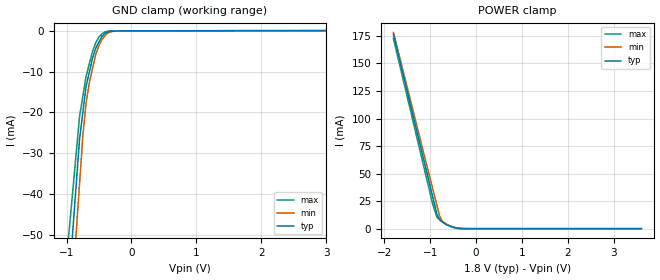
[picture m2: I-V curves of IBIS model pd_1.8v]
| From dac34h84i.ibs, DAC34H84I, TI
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[Model] pd_1.8v
Model_type Input
Vinl = 540.000mV
Vinh = 1.26000V
C_comp 1.63000pF 1.63000pF 1.63000pF
| variable typ   min   max
[Voltage Range] 1.80000V 1.70000V 1.90000V
[POWER Clamp Reference] 1.80000V 1.70000V 1.90000V
[GND Clamp Reference] 0.00000V 0.00000V 0.00000V
[Temperature Range] 25   125   -40
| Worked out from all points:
|   GND clamp passes 1 mA (typ) near -0.43 V on its own axis
|   POWER clamp passes 1 mA (typ) near -0.47 V on its own axis
[GND Clamp]
-1.8V     -242.4mA   -269.9mA   -195.7mA
-800mV    -26.7mA    -37.63mA   -21.15mA
-750mV    -20.22mA   -26.01mA   -16.21mA
-700mV    -13.73mA   -17.89mA   -11.26mA
-650mV    -10.26mA   -12.81mA   -8.173mA
-600mV    -6.781mA   -9.304mA   -5.08mA
-550mV    -4.257mA   -5.802mA   -2.937mA
-500mV    -2.753mA   -3.618mA   -1.517mA
-450mV    -1.249mA   -2.055mA   -667.8uA
-350mV    -200.6uA   -456.3uA   -72.45uA
-150mV    -15.42uA   -17.32uA   -17.32uA
3.6V      32.18uA    37.62uA    21.08uA
[POWER Clamp]
-1.8V     176.6mA    178.2mA    172.7mA
-950mV    30.08mA    37.3mA     23.19mA
-850mV    12.85mA    20.72mA    10.26mA
-800mV    8.58mA     12.43mA    8.407mA
-750mV    6.431mA    7.761mA    6.555mA
-700mV    5.13mA     5.591mA    5.214mA
-550mV    2.047mA    2.306mA    1.852mA
-300mV    100.4uA    94.42uA    51.97uA
3.6V      0A         0A         0A
